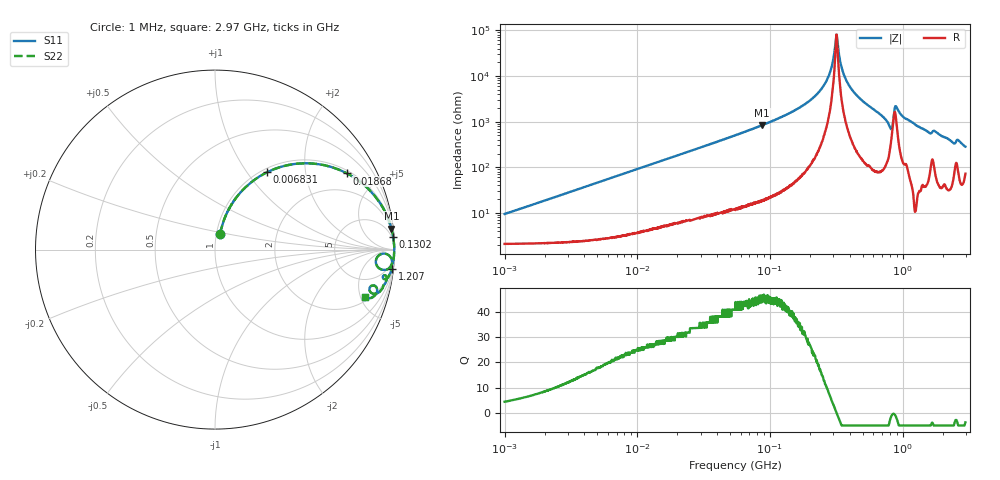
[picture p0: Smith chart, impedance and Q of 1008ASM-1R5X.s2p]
!s-Parameter Generated by FASTRON Sdn. Bhd.
!FASTRON P/N : 1008ASM-1R5X
!Keysight Technologies: E4991B_MY54100416_A.01.15
!Date: Tue Nov 21 10:00:33 2023
!Version  :Rev00  Wed Nov 22 15:06:53 2023
!Data & Calibration Information:
!Freq  S11  S21  S12  S22
!PortZ  Port1:50+j0  Port2:50+j0
!When reading reference impedance value at option line is always used.
! Remarks : This data is being provided solely for informational purposes.
# Hz S dB R 50
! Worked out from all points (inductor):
!   1599 points, 1 MHz to 2.97 GHz, reference 50 ohm
!   read as one part in series: L = 1.47 uH near 1.036 MHz
!   highest Q = 45.8 at 87.23 MHz (marker M1), where L = 1.52 uH
!   self-resonance near 317.2 MHz
!   S11 on the Smith chart (normalised r, x): 1 MHz: 1.04, +0.18; 6.831 MHz: 1.06, +1.25; 18.68 MHz: 1.11, +3.39; 130.2 MHz: 2, +28; 1.207 GHz: 1, -19; 2.97 GHz: 2.45, -5.47
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1000000  -20.70 72.1  -0.22 -5.2  -0.22 -5.2  -20.70 72.1
3804036  -9.78 67.2  -0.69 -18.9  -0.69 -18.9  -9.78 67.2
6831390  -5.67 56.0  -1.62 -31.3  -1.62 -31.3  -5.67 56.0
1.439846e7  -2.14 36.6  -4.49 -51.4  -4.49 -51.4  -2.14 36.6
1.867766e7  -1.42 30.0  -6.01 -58.0  -6.01 -58.0  -1.42 30.0
5.477226e7  -0.21 11.2  -14.20 -77.4  -14.20 -77.4  -0.21 11.2
8.723049e7  -0.08 6.8  -18.50 -81.9  -18.50 -81.9  -0.08 6.8
1.30174e8  -0.04 4.1  -22.80 -84.5  -22.80 -84.5  -0.04 4.1
2.073156e8  -0.02 1.8  -30.00 -85.8  -30.00 -85.8  -0.02 1.8
2.716345e8  -0.01 0.6  -38.90 -83.2  -38.90 -83.2  -0.01 0.6
2.898922e8  -0.01 0.4  -43.50 -79.0  -43.50 -79.0  -0.01 0.4
3.10929e8  -0.01 0.1  -54.10 -50.5  -54.10 -50.5  -0.01 0.1
3.188066e8  -0.01 -0.0  -57.80 13.8  -57.80 13.8  -0.01 -0.0
3.523638e8  -0.01 -0.4  -42.30 79.9  -42.30 79.9  -0.01 -0.4
4.013235e8  -0.01 -1.0  -35.20 84.4  -35.20 84.4  -0.01 -1.0
7.846996e8  -0.24 -6.3  -19.00 72.8  -19.00 72.8  -0.24 -6.3
8.208471e8  -0.77 -6.3  -17.40 47.8  -17.40 47.8  -0.77 -6.3
8.937307e8  -0.21 -2.3  -26.80 57.9  -26.80 57.9  -0.21 -2.3
1.01283e9  -0.09 -4.5  -22.10 80.0  -22.10 80.0  -0.09 -4.5
1.206698e9  -0.07 -6.2  -19.40 82.5  -19.40 82.5  -0.07 -6.2
1.581072e9  -0.28 -9.7  -15.40 74.5  -15.40 74.5  -0.28 -9.7
2.970126e9  -1.16 -17.4  -10.20 57.8  -10.20 57.8  -1.16 -17.4
